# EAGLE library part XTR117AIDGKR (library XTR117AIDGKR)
Sensor Interface XTR117 4-20mA Crnt Loop Transmitter Source: Datasheet
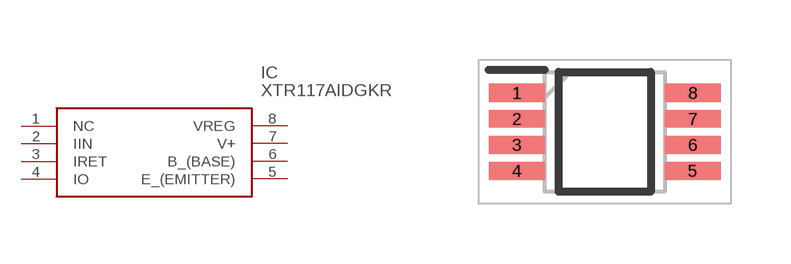
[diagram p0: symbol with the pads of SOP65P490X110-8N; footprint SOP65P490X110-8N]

Designator prefix IC

## XTR117AIDGKR (Description: Sensor Interface XTR117 4-20mA Crnt Loop Transmitter; Height: 1.1mm; Manufacturer_Name: Texas Instruments; Manufacturer_Part_Number: XTR117AIDGKR; Mouser_Part_Number: 595-XTR117AIDGKR; Mouser_Price-Stock: https://www.mouser.co.uk/ProductDetail/Texas-Instruments/XTR117AIDGKR?qs=zqbRmZ%252BfZD%252BYMdmF%252BmhQwg%3D%3D)  [SOP65P490X110-8N]
1  NC  nc
2  IIN
3  IRET
4  IO
5  E_(EMITTER)
6  B_(BASE)
7  V+
8  VREG

## Footprint SOP65P490X110-8N (pad centres in mm)
DGK (S-PDSO-G8)
smd 1.4 x 0.45: 1 -2.2,0.975; 2 -2.2,0.325; 3 -2.2,-0.325; 4 -2.2,-0.975; 5 2.2,-0.975; 6 2.2,-0.325; 7 2.2,0.325; 8 2.2,0.975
